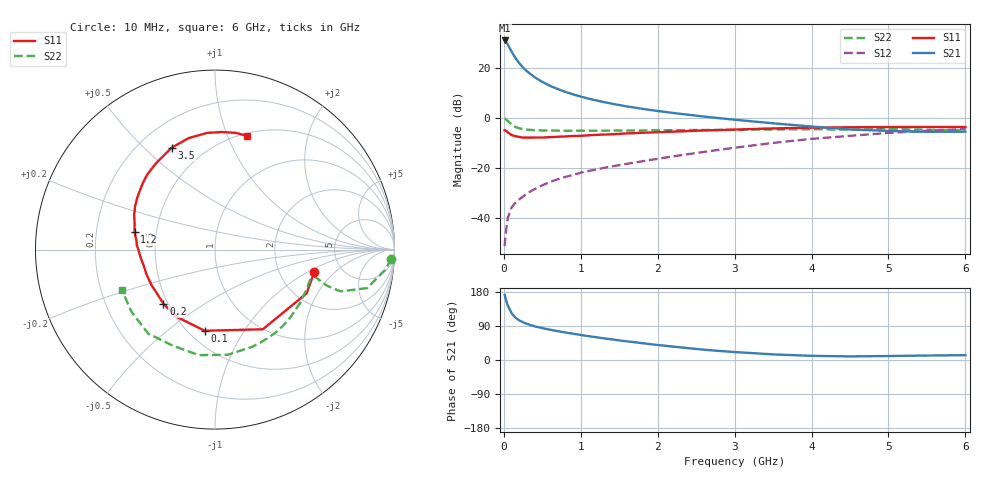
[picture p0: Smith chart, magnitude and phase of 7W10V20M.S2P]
! Infineon Technologies  Discrete & RF Semiconductors
! BFS17W
! Si NPN RF Bipolar Junction Transistor in SOT323
! VCE = 10 V  IC = 20 mA
! Common Emitter S-Parameters:  August  1999
# GHz  S  MA  R  50
!  f  S11  S21  S12  S22
! GHz  MAG  ANG  MAG  ANG  MAG  ANG  MAG  ANG
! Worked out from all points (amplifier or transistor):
!   36 points, 10 MHz to 6 GHz, reference 50 ohm
!   highest |S21| = 30.8 dB at 10 MHz (marker M1)
!   |S21| within 3 dB of that: start of sweep to 75.38 MHz
!   unconditionally stable (mu >= 1): 329.5 MHz to 1.99 GHz; 5.753 GHz to end of sweep
!   at 250 MHz: K = 0.94, MSG = 25.7 dB, |S12| = -31.3 dB
!   at 1.4 GHz: K = 1.13, MAG = 10.3 dB, |S12| = -19.4 dB
!   at 6 GHz: K = 1.02, MAG = -1.3 dB, |S12| = -4.5 dB
!   S11 on the Smith chart (normalised r, x): 10 MHz: 3.15, -1.17; 100 MHz: 0.60, -0.69; 200 MHz: 0.47, -0.35; 1.2 GHz: 0.38, +0.09; 3.5 GHz: 0.33, +0.61; 6 GHz: 0.53, +1.17
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0.01  0.5673 -12.8  34.72 171.9  0.0028 83.7  0.9841 -3.0
0.02  0.5655 -25.6  33.97 164.0  0.0044 75.7  0.9543 -6.8
0.05  0.5178 -59.0  29.08 144.4  0.01 70.3  0.8742 -14.2
0.1  0.4558 -97.1  20.88 123.8  0.0164 61.3  0.7371 -18.4
0.15  0.4314 -119.9  15.57 111.9  0.0205 58.9  0.6591 -17.9
0.2  0.4165 -133.6  12.27 104.6  0.0239 62.6  0.62 -16.9
0.25  0.4049 -143.5  10.03 99.4  0.0272 62.1  0.5969 -15.9
0.3  0.4054 -150.4  8.472 95.3  0.0313 64.5  0.5846 -15.5
0.4  0.406 -160.3  6.452 88.9  0.0383 66.3  0.5692 -15.2
0.5  0.4068 -166.9  5.198 84.1  0.0455 68.7  0.5632 -15.6
0.6  0.4135 -172.1  4.343 79.9  0.0529 69.9  0.5593 -16.4
0.7  0.4202 -176.1  3.75 76.1  0.0602 70.5  0.5568 -17.6
0.9  0.4369 176.6  2.936 69.3  0.0733 71.4  0.5546 -20.6
1.1  0.4509 170.2  2.422 62.9  0.0876 72.1  0.5561 -24.2
1.2  0.4582 167.7  2.228 60.1  0.094 72.6  0.5558 -26.1
1.6  0.4919 156.4  1.69 49.2  0.1219 73.9  0.5589 -34.5
2.2  0.5311 142.2  1.253 35.3  0.1712 75.4  0.5691 -48.7
2.8  0.5721 128.1  0.986 23.9  0.2318 74.2  0.5764 -64.1
3.5  0.6172 113.0  0.78 14.8  0.3178 69.6  0.5905 -83.1
4.5  0.6515 93.9  0.589 9.5  0.4396 57.7  0.5844 -113.9
5.5  0.6606 79.8  0.528 11.8  0.5532 44.4  0.5804 -143.3
6  0.6579 74.4  0.532 12.7  0.5986 37.7  0.5652 -156.8
